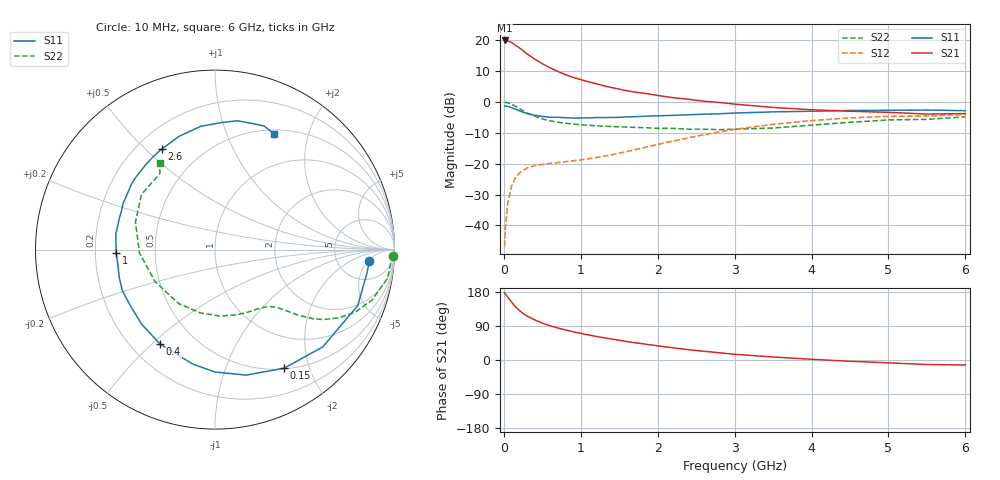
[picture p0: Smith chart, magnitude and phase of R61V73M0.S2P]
! SIEMENS Small Signal Semiconductors
! BFR193
! Si NPN RF Bipolar Junction Transistor in SOT23
! VCE = 1.75 V  IC = 3 mA
! Common Emitter S-Parameters:  May  1996
# GHz  S  MA  R  50
!  f  S11  S21  S12  S22
! GHz  MAG  ANG  MAG  ANG  MAG  ANG  MAG  ANG
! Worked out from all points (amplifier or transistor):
!   36 points, 10 MHz to 6 GHz, reference 50 ohm
!   highest |S21| = 20.0 dB at 10 MHz (marker M1)
!   |S21| within 3 dB of that: start of sweep to 234 MHz
!   unconditionally stable (mu >= 1): 1.041 GHz to 2.023 GHz
!   at 250 MHz: K = 0.31, MSG = 19.4 dB, |S12| = -22.2 dB
!   at 1.4 GHz: K = 1.10, MAG = 9.0 dB, |S12| = -17.1 dB
!   at 6 GHz: K = 0.99, MSG = 0.2 dB, |S12| = -4.1 dB
!   S11 on the Smith chart (normalised r, x): 10 MHz: 11, -5; 150 MHz: 0.51, -1.62; 400 MHz: 0.32, -0.53; 1 GHz: 0.29, -0.02; 2.6 GHz: 0.30, +0.56; 6 GHz: 0.55, +1.49
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0.01  0.862 -4.3  9.945 177.5  0.0046 86.8  0.995 -1.9
0.02  0.8569 -8.7  9.747 174.2  0.0092 86.5  0.9835 -3.7
0.05  0.8544 -21.4  9.713 165.9  0.0229 78.6  0.9751 -9.3
0.1  0.8089 -42.1  9.245 152.8  0.0429 68.4  0.92 -17.7
0.15  0.7647 -59.8  8.305 140.8  0.0588 60.2  0.8539 -24.2
0.2  0.7204 -76.1  7.586 131.1  0.0701 53.8  0.7852 -29.0
0.25  0.6819 -90.1  6.797 122.6  0.078 48.5  0.7181 -32.9
0.3  0.6494 -101.0  6.044 116.2  0.0847 45.3  0.6662 -35.3
0.4  0.609 -120.1  4.972 106.0  0.0929 40.9  0.5894 -38.3
0.5  0.5828 -134.6  4.165 97.3  0.0972 38.7  0.5311 -40.3
0.6  0.5658 -146.1  3.59 90.5  0.101 38.4  0.4943 -41.8
0.8  0.5559 -163.6  2.78 79.4  0.1078 39.7  0.4525 -44.7
1  0.5509 -177.9  2.305 70.2  0.1151 43.9  0.4279 -48.2
1.1  0.5532 176.1  2.126 66.1  0.12 46.0  0.4185 -50.6
1.3  0.5579 165.5  1.832 58.8  0.1326 50.3  0.4038 -55.2
1.6  0.5729 153.2  1.521 48.7  0.1571 55.3  0.3919 -63.7
2.2  0.6068 131.1  1.175 32.2  0.232 58.3  0.3734 -84.8
2.6  0.6342 118.0  1.03 23.0  0.2941 55.5  0.3625 -102.9
3.5  0.6915 96.5  0.817 7.9  0.4344 41.3  0.3786 -151.8
4.5  0.7285 80.2  0.708 -3.4  0.5523 22.5  0.4688 161.0
5.5  0.7412 68.3  0.638 -11.9  0.5928 4.5  0.5233 125.9
6  0.7233 63.0  0.65 -13.2  0.627 -0.6  0.5743 122.4
